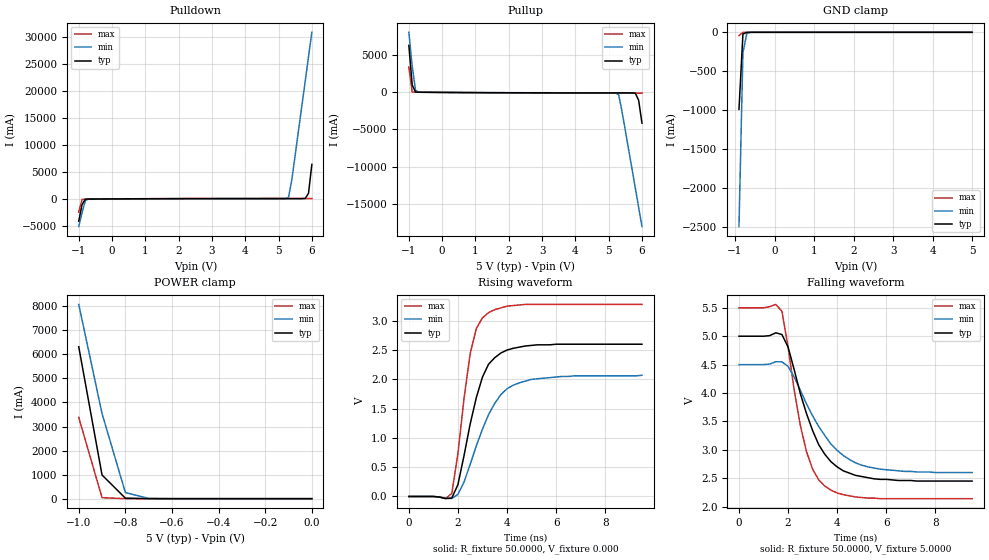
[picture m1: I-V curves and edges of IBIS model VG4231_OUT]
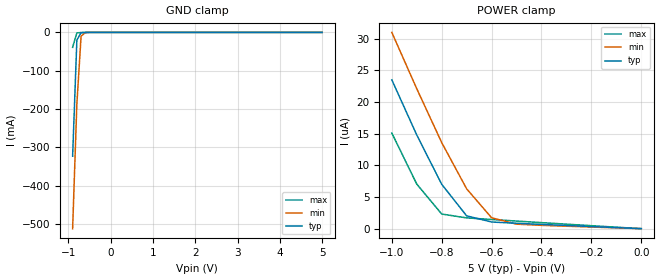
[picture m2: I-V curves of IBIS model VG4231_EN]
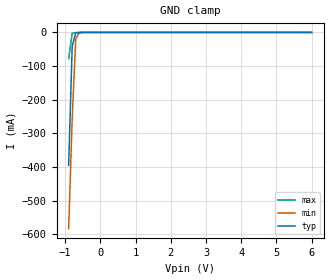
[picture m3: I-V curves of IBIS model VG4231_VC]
[IBIS ver]   2.1
[File name]   4231cahf.ibs
[File Rev]   0.1
[Date]   March 23, 2005
[Copyright]   Copyright 2005, EPSONTOYOCOM Corp.
|   Component VG4231xxH
[Component]   VG4231xxH
[Manufacturer]   EPSONTOYOCOM Corp.
[Package]
| variable   typ   min   max
R_pkg   0.20   0.13   0.28
L_pkg   5.16nH   4.56nH   5.76nH
C_pkg   1.23pF   1.03pF   1.53pF
[Pin]  signal_name   model_name   R_pin   L_pin   C_pin
1   VC   VG4231_VC
2   NC   NC
3   GND   GND
4   OUT   VG4231_OUT
5   OE   VG4231_EN
6   VDD   POWER
| Models and submodels in the file (3): VG4231_OUT (3-state), VG4231_EN (Input), VG4231_VC (Input)
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|   Model VG4231_OUT
[Model]   VG4231_OUT
Model_type   3-state
Polarity   Non-Inverting
Enable   Active-High
C_comp   2.2010pF   2.2010pF   2.2010pF
[Temperature Range]   27.0000   85.0000   -40.0000
[Voltage Range]   5.0000V   4.5000V   5.5000V
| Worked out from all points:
|   slope of the pulldown table from 0 to 0.75 V, typ, clamps not added: 32.8 ohm
|   slope of the pullup table from 0 to 0.75 V, typ, clamps not added: 35.3 ohm
|   GND clamp passes 1 mA (typ) near -0.70 V on its own axis
|   POWER clamp passes 1 mA (typ) near -0.70 V on its own axis
|   rising waveform, R_fixture 50.0000, V_fixture 0.000: 20-80 % time 886ps typ, 1.22ns min, 636ps max; typ from 0 V to 2.6 V
|   falling waveform, R_fixture 50.0000, V_fixture 5.0000: 20-80 % time 1.24ns typ, 1.6ns min, 885ps max; typ from 5 V to 2.45 V
[Pulldown]
| voltage   I(typ)   I(min)   I(max)
-1V       -4.11A     -5.11A     -2.45A
-900mV    -1.02A     -2.52A     -82.8mA
-800mV    -49.2mA    -281mA     -37.5mA
-700mV    -24.8mA    -29.1mA    -32.6mA
5.1V      57.2mA     42mA       79.1mA
5.2V      57.3mA     52.1mA     79.1mA
5.3V      57.3mA     296mA      79.1mA
5.4V      57.3mA     3.58A      79.2mA
5.8V      79mA       21.7A      79.4mA
5.9V      1.04A      26.3A      79.4mA
6V        6.38A      30.8A      79.5mA
[Pullup]
| voltage   I(typ)   I(min)   I(max)
-1V       6.35A      8.11A      3.42A
-900mV    1.01A      3.57A      78.4mA
-800mV    47.6mA     276mA      34.2mA
-700mV    23.7mA     29.5mA     29.5mA
5.1V      -68.7mA    -52.6mA    -93mA
5.2V      -68.9mA    -62.9mA    -93.2mA
5.3V      -69.1mA    -313mA     -93.4mA
5.4V      -69.2mA    -2.55A     -93.6mA
5.8V      -92.1mA    -12.9A     -94.3mA
5.9V      -1.06A     -15.5A     -94.5mA
6V        -4.15A     -18.1A     -94.7mA
[GND_clamp]
| voltage   I(typ)   I(min)   I(max)
-900mV    -988mA     -2.49A     -42.8mA
-800mV    -22.3mA    -261mA     -1.3mA
-700mV    -968uA     -10.8mA    -315uA
-500mV    -14.7uA    -62uA      -1.68uA
5V        113pA      95.8uA     93pA
[POWER_clamp]
| voltage   I(typ)   I(min)   I(max)
-1V       6.32A      8.08A      3.38A
-900mV    985mA      3.54A      40.6mA
-800mV    21.5mA     254mA      540uA
-700mV    770uA      10.7mA     43.6uA
-600mV    84.6uA     712uA      4.3uA
-500mV    10.8uA     95.8uA     259nA
-400mV    1.01uA     13.7uA     7.74nA
-300mV    59.4nA     1.55uA     282pA
-200mV    2.52nA     124nA      134pA
-100mV    191pA      7.24nA     127pA
0V        113pA      229pA      121pA
[Ramp]
| variable   typ   min   max
dV/dt_r   1.56/0.868n   1.24/1.21n   1.97/0.605n
dV/dt_f   1.53/1.25n   1.14/1.60n   2.02/0.846n
R_load = 50.0000
[Rising Waveform]
R_fixture = 50.0000
V_fixture = 0.000
V_fixture_min = 0.000
V_fixture_max = 0.000
| time   V(typ)   V(min)   V(max)
0s        3.17nV     15.8nV     3.44nV
1.75ns    -27mV      -34.9mV    52.2mV
2ns       203mV      35.9mV     735mV
2.25ns    701mV      247mV      1.68V
2.5ns     1.24V      551mV      2.44V
2.75ns    1.69V      866mV      2.87V
3.25ns    2.26V      1.4V       3.14V
4ns       2.5V       1.84V      3.25V
5ns       2.58V      2V         3.28V
9.5ns     2.6V       2.07V      3.28V
[Falling Waveform]
R_fixture = 50.0000
V_fixture = 5.0000
V_fixture_min = 4.5000
V_fixture_max = 5.5000
| time   V(typ)   V(min)   V(max)
0s        5V         4.5V       5.5V
1.5ns     5.06V      4.55V      5.56V
1.75ns    5.03V      4.55V      5.44V
2ns       4.81V      4.47V      4.81V
2.5ns     3.99V      4.05V      3.43V
2.75ns    3.64V      3.81V      2.97V
3.5ns     2.92V      3.25V      2.36V
4.25ns    2.63V      2.9V       2.21V
5.25ns    2.51V      2.7V       2.15V
9.5ns     2.45V      2.6V       2.14V
|   Model VG4231_EN
[Model]   VG4231_EN
Model_type   Input
Vinl =   1.0000V
Vinh =   4.0000V
C_comp   1.4070pF   1.4070pF   1.4070pF
[Temperature Range]   27.0000   85.0000   -40.0000
[Voltage Range]   5.0000V   4.5000V   5.5000V
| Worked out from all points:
|   GND clamp passes 1 mA (typ) near -0.70 V on its own axis
[GND_clamp]
| voltage   I(typ)   I(min)   I(max)
-900mV    -323mA     -512mA     -39mA
-800mV    -20.3mA    -187mA     -1.24mA
-700mV    -918uA     -9.88mA    -315uA
-600mV    -141uA     -601uA     -41.7uA
5V        27.5pA     712nA      25pA
[POWER_clamp]
| voltage   I(typ)   I(min)   I(max)
-1V       23.5uA     31uA       15.1uA
-900mV    14.8uA     22.1uA     7.04uA
-800mV    7.01uA     13.6uA     2.31uA
-700mV    2.02uA     6.29uA     1.7uA
-600mV    1.05uA     1.72uA     1.45uA
-500mV    851nA      712nA      1.2uA
-400mV    674nA      526nA      953nA
-300mV    501nA      388nA      709nA
-200mV    331nA      256nA      469nA
-100mV    164nA      126nA      233nA
0V        27.5pA     152pA      27.5pA
|   Model VG4231_VC
[Model]   VG4231_VC
Model_type   Input
Vinl =   1.000V
Vinh =   4.000V
C_comp   1.4070pF   1.4070pF   1.4070pF
[Temperature Range]   27.0000   85.0000   -40.0000
[Voltage Range]   5.0000V   4.5000V   5.5000V
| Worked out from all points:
|   GND clamp passes 1 mA (typ) near -0.65 V on its own axis
[GND_clamp]
| voltage   I(typ)   I(min)   I(max)
-900mV    -395mA     -583mA     -77.7mA
-800mV    -40.6mA    -257mA     -2.48mA
-700mV    -1.84mA    -19.7mA    -632uA
-600mV    -282uA     -1.2mA     -81.5uA
6V        50uA       42.9uA     60uA
